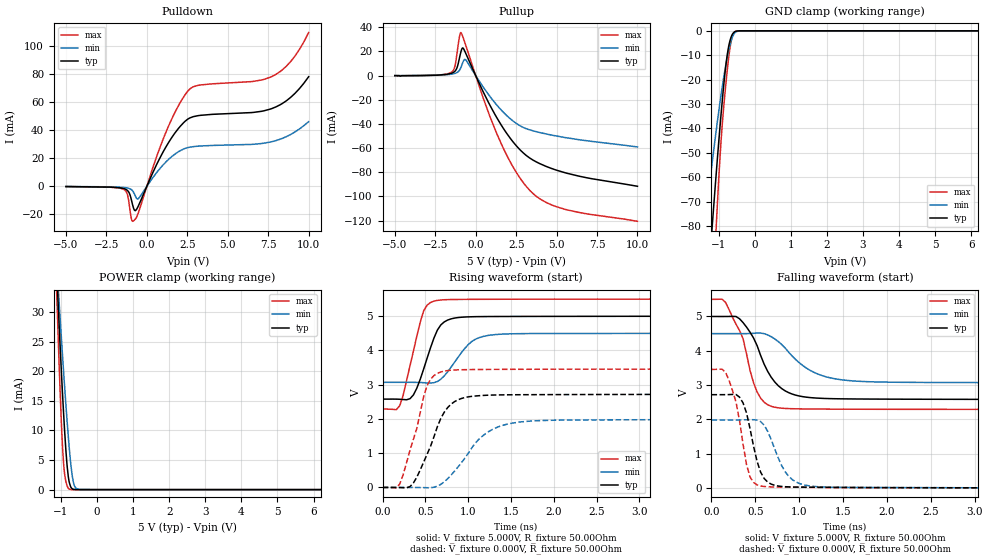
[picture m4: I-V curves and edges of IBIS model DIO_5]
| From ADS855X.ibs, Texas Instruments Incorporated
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|   I/O 5.0V Model
[Model]   DIO_5
Model_type   I/O
|Polarity   Non-Inverting
Enable   Active-High
Vinl = -300.000mV   |min, BGND -0.3V
Vinh = 5.8V   |max. BVDD +0.3V
Vmeas = 2.385V
Cref = 30.00pF
Rref = 82   |For BVDD=2.7 [{0.3*BVDD/Imax}-Rout(max) with Imax=5mA, Rout_max=80ohm]
|Signals   DB14/REFBUFEN, DB13/SDI, DB12, DB11, DB10/SDO_C, DB9/SDO_B
|   DB8/SDO_A, DB7/HBEN/DCEN, DB6/SCLK, DB5/DCIN_A, DB4/DCIN_B,
|   DB3/DCIN_C, DB2/SEL_C, DB1/SEL_B, DB0/SEL_A, RANGE/XCLK,
|   DB15
| C_comp   obtained at 25MHz
| variable   typ   min   max
|C_comp Output Disable
C_comp   3.385pF   2.581pF   4.140pF
|C_comp Output Low
|C_comp   3.602pF   2.835pF   4.383pF
|C_comp Output High
|C_comp   3.748pF   2.959pF   4.677pF
[Model Spec]
|Timing spec test load voltage corners 0.5*VCC
|  To be verified
Vmeas   2.39V   2.20V   2.68V
Vref   2.50V   0.50V   3.00V
|Junction Temperature
[Temperature Range]   40.0   125.0   -40.0
[Voltage range]   5.0V   4.50V   5.50V
[pullup reference]   5.0V   4.50V   5.50V
[power clamp reference]   5.0V   4.50V   5.50V
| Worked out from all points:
|   slope of the pulldown table from 0 to 0.75 V, typ, clamps not added: 39.6 ohm
|   slope of the pullup table from 0 to 0.75 V, typ, clamps not added: 35.6 ohm
|   GND clamp passes 1 mA (typ) near -0.60 V on its own axis
|   POWER clamp passes 1 mA (typ) near -0.76 V on its own axis
|   falling waveform, V_fixture 5.000V, R_fixture 50.00Ohm: 20-80 % time 285ps typ, 395ps min, 236ps max; typ from 5 V to 2.58 V
|   rising waveform, V_fixture 5.000V, R_fixture 50.00Ohm: 20-80 % time 201ps typ, 268ps min, 181ps max; typ from 2.58 V to 5 V
|   rising waveform, V_fixture 0.000V, R_fixture 50.00Ohm: 20-80 % time 270ps typ, 399ps min, 217ps max; typ from 0 V to 2.72 V
|   falling waveform, V_fixture 0.000V, R_fixture 50.00Ohm: 20-80 % time 148ps typ, 211ps min, 150ps max; typ from 2.72 V to 0 V
[Pulldown]
|   Voltage   I(typ)   I(min)   I(max)
-5V       -197.3uA   -142.6uA   -199.2uA
-1.436V   -1.615mA   -846uA     -2.197mA
-1.205V   -2.944mA   -1.242mA   -5.731mA
-972.5mV  -8.952mA   -2.284mA   -22.44mA
-822.5mV  -15.68mA   -4.262mA   -24.69mA
-524.4mV  -13.98mA   -8.842mA   -18.82mA
600.6mV   15.5mA     9.755mA    21.13mA
1.308V    30.67mA    18.86mA    42.2mA
2.635V    48.76mA    27.94mA    69.39mA
7.741V    55.68mA    31.96mA    78.62mA
8.914V    63.91mA    37.25mA    89.64mA
9.998V    78.4mA     46.21mA    110mA
[GND Clamp]
|   Voltage   I(typ)   I(min)   I(max)
-5V       -965.7mA   -668.8mA   -1.352A
-1.402V   -126.5mA   -82.34mA   -183.3mA
-1.312V   -107.4mA   -70.57mA   -154.8mA
-1.166V   -77.55mA   -52.34mA   -109.4mA
-1.094V   -63.6mA    -43.91mA   -88.07mA
-1.053V   -55.75mA   -39.19mA   -76.11mA
-968.8mV  -40.35mA   -29.96mA   -53.42mA
-914.4mV  -31.04mA   -24.37mA   -41.2mA
-771.9mV  -10.89mA   -11.62mA   -17.61mA
-651.9mV  -2.469mA   -4.02mA    -4.15mA
-522.5mV  -179.9uA   -465.9uA   -188.1uA
9.998V    68.2nA     87.7nA     48.86nA
[Pullup]
|   Voltage   I(typ)   I(min)   I(max)
-5V       -23.11uA   -8.477uA   -39.1uA
-1.511V   1.862mA    1.137mA    2.667mA
-1.278V   3.689mA    1.83mA     7.96mA
-1.012V   13.94mA    4.245mA    31.42mA
-918.1mV  19.39mA    6.527mA    35.61mA
-792.5mV  22.86mA    10.95mA    32.06mA
-618.1mV  18.56mA    13.09mA    25.21mA
1.371V    -36.33mA   -25.38mA   -50.05mA
2.311V    -54.86mA   -37.58mA   -75.62mA
3.333V    -68.13mA   -44.87mA   -94.79mA
5.472V    -80.17mA   -51.13mA   -110.5mA
9.998V    -91.57mA   -59.05mA   -120.6mA
[POWER Clamp]
|   Voltage   I(typ)   I(min)   I(max)
-5V       320.7mA    274.7mA    381.2mA
-1.117V   36.27mA    38.08mA    32.47mA
-1.055V   28.03mA    31.85mA    21.43mA
-1.001V   21.14mA    26.56mA    12.71mA
-953.8mV  15.6mA     22.17mA    6.678mA
-914.4mV  11.3mA     18.6mA     3.371mA
-869.4mV  6.963mA    14.67mA    1.459mA
-828.1mV  3.801mA    11.25mA    561.2uA
-770mV    1.186mA    6.872mA    84.49uA
-657.5mV  45.3uA     1.24mA     2.004uA
-485mV    108nA      12.27uA    43.95nA
9.998V    -55.4nA    -67.77nA   -43.39nA
[Ramp]
R_load = 50.00Ohm
|   typ   min   max
dV/dt_r   1.631V/270.076ps   1.188V/398.602ps   2.074V/217.348ps
dV/dt_f   1.452V/284.745ps 858.201mV/394.568ps   1.926V/236.177ps
[Falling Waveform]
V_fixture = 5.000V
V_fixture_min = 4.500V
V_fixture_max = 5.500V
R_fixture = 50.00Ohm
|   Time   V(typ)   V(min)   V(max)
0s        5V         4.5V       5.5V
160ps     5V         4.5V       5.413V
320ps     4.933V     4.499V     4.59V
360ps     4.822V     4.499V     4.352V
520ps     4.15V      4.515V     2.8V
680ps     3.229V     4.411V     2.38V
920ps     2.736V     3.844V     2.309V
1.16ns    2.626V     3.38V      2.3V
1.44ns    2.599V     3.168V     2.296V
4ns       2.58V      3.07V      2.289V
[Rising Waveform]
V_fixture = 5.000V
V_fixture_min = 4.500V
V_fixture_max = 5.500V
R_fixture = 50.00Ohm
|   Time   V(typ)   V(min)   V(max)
0s        2.58V      3.07V      2.289V
200ps     2.576V     3.07V      2.388V
360ps     2.702V     3.069V     3.985V
480ps     3.463V     3.06V      5.159V
600ps     4.365V     3.06V      5.442V
680ps     4.747V     3.161V     5.475V
760ps     4.889V     3.379V     5.486V
1ns       4.982V     4.17V      5.493V
1.24ns    4.992V     4.442V     5.496V
4ns       5V         4.5V       5.5V
[Rising Waveform]
V_fixture = 0.000V
V_fixture_min = 0.000V
V_fixture_max = 0.000V
R_fixture = 50.00Ohm
|   Time   V(typ)   V(min)   V(max)
0s        -1.322uV   -2.137uV   -813.2nV
200ps     -2.862mV   232.9uV    101.3mV
360ps     132mV      46.69uV    1.409V
520ps     971.3mV    -8.564mV   2.976V
680ps     2.016V     90.37mV    3.372V
800ps     2.433V     360.2mV    3.424V
920ps     2.598V     720.4mV    3.438V
1.16ns    2.685V     1.487V     3.446V
1.48ns    2.706V     1.861V     3.45V
4ns       2.718V     1.981V     3.456V
[Falling Waveform]
V_fixture = 0.000V
V_fixture_min = 0.000V
V_fixture_max = 0.000V
R_fixture = 50.00Ohm
|   Time   V(typ)   V(min)   V(max)
0s        2.718V     1.981V     3.456V
160ps     2.719V     1.981V     3.377V
280ps     2.723V     1.981V     2.502V
320ps     2.646V     1.982V     1.957V
400ps     2.183V     1.987V     673.9mV
520ps     770.4mV    1.976V     86.09mV
680ps     109.4mV    1.411V     27.9mV
840ps     33.4mV     467.8mV    21.16mV
1.08ns    20.04mV    72.64mV    14.28mV
4ns       -1.322uV   -2.137uV   -813.2nV
